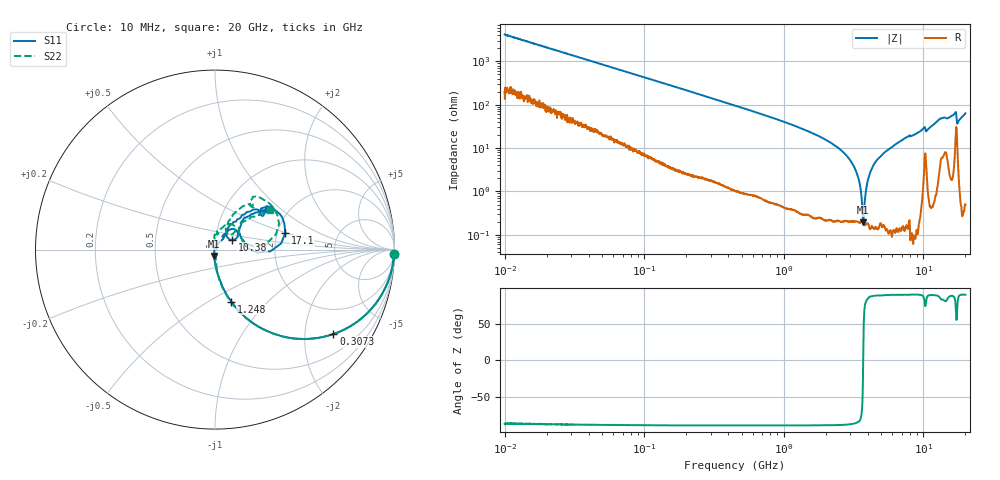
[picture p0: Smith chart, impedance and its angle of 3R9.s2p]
!Keysight Technologies,P5008B,MY61100088,A.16.20.02
!Date: Friday, August 30, 2024 12:56:13
!Correction: S11(C  2-Port  )
!S21(C  2-Port  )
!S12(C  2-Port  )
!S22(C  2-Port  )
!S2P File: Measurements: S11, S21, S12, S22:Log Frequency Sweep
# Hz S  dB  R 50
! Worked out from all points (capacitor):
!   1601 points, 10 MHz to 20 GHz, reference 50 ohm
!   read as one part in series: C = 3.84 pF near 10.39 MHz
!   lowest |Z| = 196 mohm at 3.704 GHz (marker M1)
!   series resonance near 3.704 GHz, so ESL is about 480 pH
!   S11 on the Smith chart (normalised r, x): 10 MHz: 3, -82; 307.3 MHz: 1.02, -2.79; 1.248 GHz: 1.00, -0.64; 10.38 GHz: 1.20, +0.13; 17.1 GHz: 2.21, +0.49; 20 GHz: 1.58, +0.83
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1e7  -0.01 -1.4  -32.39 85.9  -32.38 86.0  -0.01 -1.4
3.555162e7  -0.05 -4.8  -21.54 83.4  -21.54 83.4  -0.05 -4.8
1.263918e8  -0.40 -16.5  -11.02 72.7  -11.03 72.7  -0.39 -16.5
3.072746e8  -1.83 -35.5  -4.79 53.8  -4.79 53.8  -1.83 -35.5
4.472136e8  -3.24 -46.2  -2.89 43.1  -2.89 43.1  -3.23 -46.3
1.247826e9  -10.34 -72.5  -0.45 16.6  -0.45 16.6  -10.34 -73.2
1.589917e9  -12.77 -77.4  -0.26 11.8  -0.26 11.8  -12.76 -77.8
2.771802e9  -20.28 -87.7  -0.06 2.5  -0.06 2.5  -20.17 -84.6
3.703514e9  -29.05 -97.6  -0.02 -2.0  -0.02 -2.1  -28.43 -79.8
4.053346e9  -34.47 -101.9  -0.01 -3.5  -0.01 -3.6  -33.66 -74.5
4.4999e9  -48.22 -179.5  -0.01 -5.3  -0.01 -5.3  -42.57 -9.5
5.263645e9  -34.51 89.3  -0.01 -8.0  -0.01 -8.0  -33.48 62.2
5.652411e9  -31.98 75.5  -0.00 -9.2  -0.00 -9.3  -31.21 76.9
7.410252e9  -21.44 55.1  -0.02 -14.9  -0.02 -15.0  -21.56 89.9
8.545299e9  -21.21 59.2  -0.02 -18.3  -0.02 -18.4  -21.23 79.8
1.038284e10  -19.27 29.3  -0.58 -22.0  -0.58 -22.1  -17.61 41.3
1.083639e10  -17.69 59.1  -0.11 -24.2  -0.11 -24.4  -17.57 62.9
1.348308e10  -9.70 40.4  -0.88 -34.0  -0.89 -34.2  -9.97 50.3
1.646043e10  -8.20 36.6  -0.89 -42.8  -0.89 -42.9  -8.34 49.0
1.709804e10  -7.91 13.3  -2.44 -43.3  -2.44 -43.5  -8.30 21.9
1.801527e10  -13.64 45.7  -0.30 -39.9  -0.30 -40.1  -13.55 45.2
2e10  -8.58 37.1  -0.66 -52.9  -0.66 -53.1  -8.48 35.4
